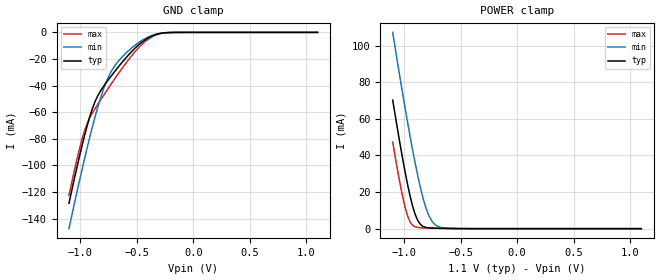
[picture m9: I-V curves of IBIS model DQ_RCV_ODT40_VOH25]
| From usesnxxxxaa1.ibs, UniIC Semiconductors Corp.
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|   Model DQ_RCV_ODT40_VOH25
[Model] DQ_RCV_ODT40_VOH25
Model_type Input
Polarity   Non-Inverting
Vinl =  0.113V
Vinh =  0.253V
C_comp   1.110pF   1.087pF   1.118pF
[Model Spec]
Vinh   0.253V   0.247V   0.265V
Vinl   0.113V   0.107V   0.125V
[Add Submodel]
|  Submodel_name   Mode
ODT40_VOH25   Non-Driving
[Temperature Range]   25.000   0.125k   -40.000
[Voltage Range]   1.100V   1.060V   1.170V
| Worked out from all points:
|   GND clamp passes 1 mA (typ) near -0.30 V on its own axis
|   POWER clamp passes 1 mA (typ) near -0.82 V on its own axis
[GND_clamp]
|Voltage   I(typ)   I(min)   I(max)
-1.1V     -128.5mA   -147.6mA   -122.6mA
-1.008V   -93.62mA   -112mA     -87.95mA
-962mV    -77.6mA    -95.05mA   -73.96mA
-893mV    -57.36mA   -71.21mA   -60.7mA
-847mV    -48.01mA   -56.81mA   -54.36mA
-801mV    -41.47mA   -44.23mA   -48.33mA
-755mV    -36.02mA   -34.19mA   -42.41mA
-709mV    -30.9mA    -26.94mA   -36.63mA
-525mV    -12.67mA   -10.3mA    -15.49mA
-387mV    -3.615mA   -3.065mA   -4.419mA
-249mV    -281uA     -330.6uA   -301.3uA
1.1V      0A         0A         0A
[POWER_clamp]
|Voltage   I(typ)   I(min)   I(max)
-1.1V     70.27mA    107.3mA    47.25mA
-1.039V   47.68mA    83.93mA    25.86mA
-993mV    31.88mA    66.94mA    12.35mA
-970mV    24.65mA    58.72mA    7.262mA
-947mV    18.06mA    50.74mA    3.761mA
-901mV    7.73mA     35.71mA    987.1uA
-855mV    2.348mA    22.46mA    514uA
-809mV    697.3uA    11.94mA    396.5uA
-763mV    321uA      5.097mA    322.7uA
-717mV    213.8uA    1.813mA    258.1uA
-556mV    65.24uA    79.15uA    81.64uA
1.1V      0A         0A         0A
